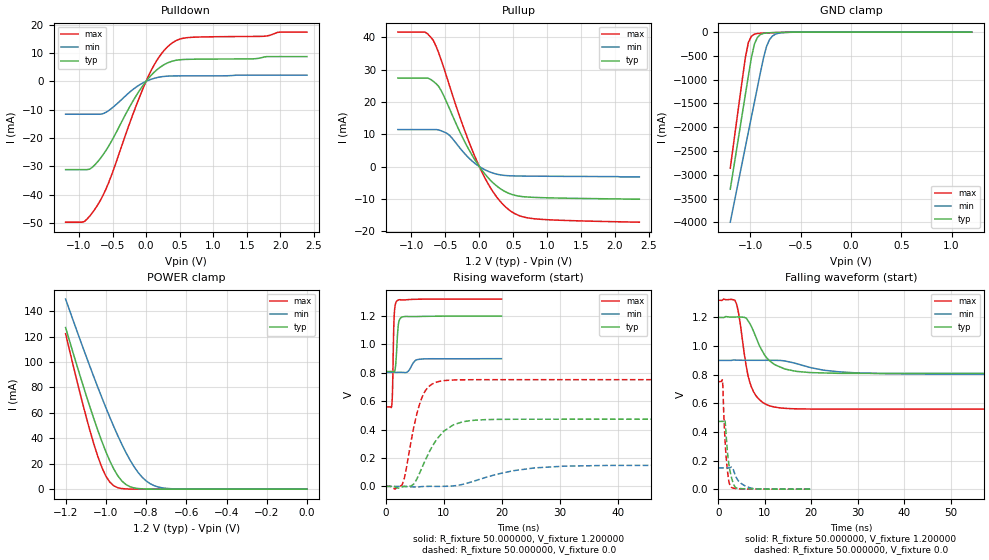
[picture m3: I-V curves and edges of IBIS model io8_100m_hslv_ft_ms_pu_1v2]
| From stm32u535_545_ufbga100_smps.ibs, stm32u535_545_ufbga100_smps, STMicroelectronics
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|   Model io8_100m_hslv_ft_ms_pu_1v2
[Model]  io8_100m_hslv_ft_ms_pu_1v2
Model_type I/O
Polarity   Non-Inverting
Enable   Active-Low
Vinl =   0.360000V
Vinh =   0.840000V
Vmeas =  0.600000V
Cref =   50.000000pF
Rref =   100.000000M
Vref =   0.0V
C_comp   3.030100pF   2.960800pF   3.078300pF
[Temperature Range]   25.000000   0.140000k   -40.000000
[Pullup Reference]   1.200000V   0.900000V   1.320000V
[Pulldown Reference]   0.0V   0.0V   0.0V
[POWER Clamp Reference]   1.200000V   0.900000V   1.320000V
[GND Clamp Reference]   0.0V   0.0V   0.0V
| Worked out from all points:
|   slope of the pulldown table from 0 to 0.18 V, typ, clamps not added: 40.7 ohm
|   slope of the pullup table from 0 to 0.18 V, typ, clamps not added: 39.5 ohm
|   GND clamp passes 1 mA (typ) near -0.51 V on its own axis
|   POWER clamp passes 1 mA (typ) near -0.86 V on its own axis
|   rising waveform, R_fixture 50.000000, V_fixture 1.200000: 20-80 % time 355ps typ, 868ps min, 231ps max; typ from 0.809 V to 1.2 V
|   rising waveform, R_fixture 50.000000, V_fixture 0.0: 20-80 % time 3.94ns typ, 8.94ns min, 2.36ns max; typ from 0.001 V to 0.474 V
|   falling waveform, R_fixture 50.000000, V_fixture 1.200000: 20-80 % time 4.09ns typ, 8.69ns min, 2.49ns max; typ from 1.2 V to 0.809 V
|   falling waveform, R_fixture 50.000000, V_fixture 0.0: 20-80 % time 1.05ns typ, 1.97ns min, 802ps max; typ from 0.474 V to 0.001 V
[Pulldown]
|Voltage   I(typ)   I(min)   I(max)
-1.2V     -31.16mA   -11.61mA   -49.71mA
-920mV    -31.16mA   -11.61mA   -49.49mA
-840mV    -31mA      -11.61mA   -47.54mA
-720mV    -28.32mA   -11.61mA   -43.58mA
-560mV    -22.95mA   -10.37mA   -35.89mA
-200mV    -7.146mA   -2.964mA   -11.89mA
0V        0A         0A         0A
160mV     4.047mA    1.298mA    7.361mA
360mV     6.869mA    1.87mA     13mA
640mV     7.765mA    1.923mA    15.46mA
1.76V     8.563mA    2.178mA    15.9mA
2.4V      8.725mA    2.178mA    17.37mA
[Pullup]
|Voltage   I(typ)   I(min)   I(max)
-1.2V     27.42mA    11.47mA    41.66mA
-800mV    27.42mA    11.47mA    41.66mA
-680mV    26.42mA    11.47mA    39.16mA
-560mV    23.45mA    11.05mA    32.89mA
-440mV    17.97mA    9.692mA    25.09mA
-200mV    7.069mA    3.643mA    10.26mA
0V        580fA      234pA      10fA
200mV     -4.978mA   -2.01mA    -7.739mA
440mV     -8.335mA   -2.843mA   -13.44mA
600mV     -9.206mA   -2.931mA   -15.29mA
840mV     -9.571mA   -2.98mA    -16.23mA
2.36V     -10.1mA    -3.2mA     -17.23mA
[GND_clamp]
|Voltage   I(typ)   I(min)   I(max)
-1.2V     -3.305A    -3.998A    -2.862A
-1.05V    -1.316A    -2.418A    -539.3mA
-1.02V    -921mA     -2.103A    -218.8mA
-990mV    -539.5mA   -1.788A    -87.43mA
-960mV    -252.1mA   -1.474A    -44.36mA
-930mV    -110.5mA   -1.16A     -30.32mA
-870mV    -28.03mA   -549.1mA   -21.09mA
-840mV    -18.43mA   -305.6mA   -18.27mA
-810mV    -13.9mA    -159.7mA   -15.73mA
-780mV    -11.23mA   -82.35mA   -13.37mA
-600mV    -2.976mA   -4.272mA   -3.058mA
1.2V      0A         14.73nA    0A
[POWER_clamp]
|Voltage   I(typ)   I(min)   I(max)
-1.2V     127mA      149.4mA    122.2mA
-1.12V    84.98mA    114mA      70.29mA
-1.06V    55.52mA    88.42mA    35.69mA
-1.02V    37.64mA    72.04mA    17.19mA
-1V       29.52mA    64.13mA    10.33mA
-960mV    15.7mA     48.99mA    2.596mA
-900mV    3.636mA    28.77mA    207.8uA
-840mV    502.9uA    13.24mA    43.56uA
-800mV    129uA      6.535mA    43.56uA
-740mV    25.39uA    1.726mA    43.56uA
-620mV    25.22uA    82.33uA    36.06uA
0V        0A         17.33nA    0A
[Ramp]
| variable   typ   min   max
dV/dt_r  0.28390/3.92634n   89.00984m/8.93147n  0.45094/2.35108n
dV/dt_f  0.23435/4.07678n   57.85200m/8.67884n  0.45609/2.47767n
R_load = 50.000000
[Rising Waveform]
R_fixture= 50.000000
V_fixture= 1.200000
V_fixture_min= 0.900000
V_fixture_max= 1.320000
|time   V(typ)   V(min)   V(max)
0s        809.5mV    803.6mV    559.9mV
1.041ns   809.9mV    803.6mV    579.2mV
1.161ns   809.6mV    803.6mV    695.3mV
1.321ns   807.4mV    803.7mV    1.051V
1.441ns   805.7mV    803.7mV    1.205V
1.922ns   1.007V     803.7mV    1.308V
2.242ns   1.16V      803.8mV    1.314V
2.923ns   1.194V     803.5mV    1.314V
5.726ns   1.197V     895.6mV    1.319V
19.94ns   1.2V       900mV      1.32V
[Rising Waveform]
R_fixture= 50.000000
V_fixture= 0.0
V_fixture_min= 0.0
V_fixture_max= 0.0
|time   V(typ)   V(min)   V(max)
0s        591.7uV    600.3uV    545.2uV
2.803ns   -2.911mV   654.4uV    10.1mV
3.203ns   113.3uV    635.5uV    59.93mV
4.805ns   16.84mV    -3.452mV   415.2mV
6.406ns   149.1mV    -323.1uV   643.9mV
8.008ns   282.4mV    762.6uV    721.9mV
10.41ns   400.6mV    1.236mV    746.9mV
15.22ns   466mV      37.75mV    751.9mV
30.83ns   473.6mV    142.9mV    752.1mV
199.4ns   473.8mV    149mV      752.2mV
[Falling Waveform]
R_fixture= 50.000000
V_fixture= 1.200000
V_fixture_min= 0.900000
V_fixture_max= 1.320000
|time   V(typ)   V(min)   V(max)
0s        1.2V       900mV      1.32V
3.604ns   1.203V     902.5mV    1.321V
4.004ns   1.204V     901.9mV    1.288V
6.406ns   1.177V     900.8mV    792.4mV
7.608ns   1.102V     900.9mV    680.1mV
10.01ns   934.5mV    900.9mV    597.3mV
13.21ns   855.2mV    900.1mV    568.7mV
22.82ns   812.3mV    831.2mV    560mV
35.24ns   809.5mV    807.7mV    559.9mV
199.4ns   809.5mV    803.6mV    559.9mV
[Falling Waveform]
R_fixture= 50.000000
V_fixture= 0.0
V_fixture_min= 0.0
V_fixture_max= 0.0
|time   V(typ)   V(min)   V(max)
0s        473.8mV    149mV      752.2mV
920.9ps   474.1mV    149.1mV    761mV
1.201ns   475.6mV    149.1mV    524.9mV
1.441ns   483mV      149.1mV    361.1mV
1.682ns   391.9mV    149.2mV    237.9mV
2.242ns   185.7mV    149mV      65.38mV
2.723ns   99.96mV    153.6mV    16.08mV
3.764ns   12.06mV    90.71mV    5.234mV
6.767ns   2.594mV    10.81mV    1.172mV
19.94ns   591.7uV    600.3uV    545.2uV
